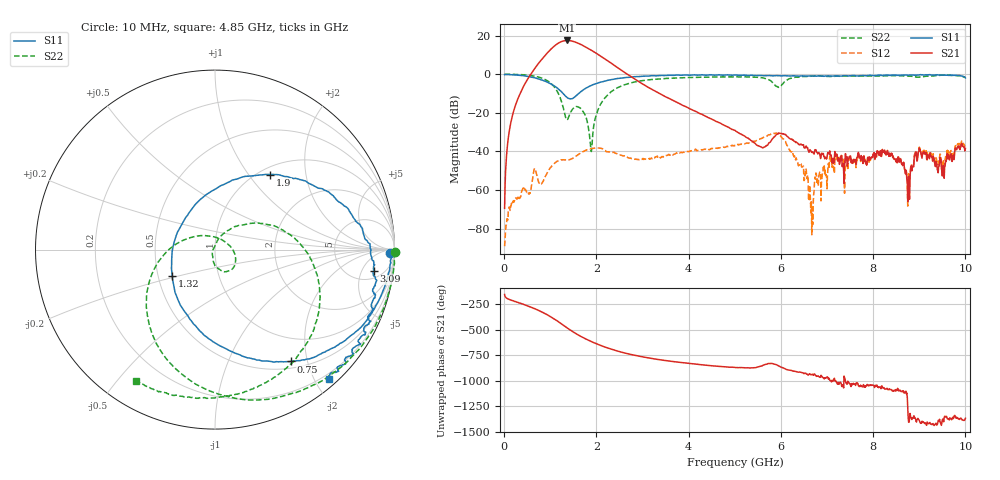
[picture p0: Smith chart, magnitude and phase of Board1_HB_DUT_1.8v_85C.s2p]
! Created Tue May 27 14:05:51 2025
# hz S ma R 50
! 2 Port Network Data from SP1.SP block
! freq  magS11  angS11  magS21  angS21  magS12  angS12  magS22  angS22
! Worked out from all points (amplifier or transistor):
!   1000 points, 10 MHz to 10 GHz, reference 50 ohm
!   highest |S21| = 17.5 dB at 1.36 GHz (marker M1)
!   |S21| within 3 dB of that: 1.083 GHz to 1.738 GHz (654.7 MHz wide, 46.4 % of centre)
!   unconditionally stable (mu >= 1): 58.74 MHz to 62.22 MHz; 90.51 MHz to 103.4 MHz; 116.1 MHz to end of sweep
!   at 1.67 GHz: K = 7.98, MAG = 16.0 dB, |S12| = -40.7 dB
!   at 5.01 GHz: K = 20.73, MAG = -12.3 dB, |S12| = -36.9 dB
!   at 10 GHz: K = 327.95, MAG = -28.9 dB, |S12| = -37.0 dB
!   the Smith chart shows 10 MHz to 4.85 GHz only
!   S11 on the Smith chart (normalised r, x): 10 MHz: 52, -44; 750 MHz: 0.60, -1.72; 1.32 GHz: 0.59, -0.19; 1.9 GHz: 1.12, +1.28; 3.09 GHz: 7, -9; 4.85 GHz: 0.12, -2.21
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1e7  0.978 -1.1  0.0003363 -153.0  3.516e-05 -168.1  1.005 -0.8
2e8  0.9631 -13.9  0.1046 145.3  0.0005206 73.5  0.9955 -18.4
7.5e8  0.7527 -55.9  1.932 50.2  0.001561 69.5  0.8425 -80.9
9.3e8  0.6291 -73.4  3.508 9.9  0.002721 115.5  0.685 -110.6
1.09e9  0.4969 -94.2  5.38 -33.2  0.004883 101.5  0.4638 -145.4
1.22e9  0.3711 -119.8  6.817 -73.2  0.005967 84.6  0.236 175.8
1.32e9  0.2793 -148.5  7.422 -105.3  0.006048 76.4  0.08705 118.4
1.36e9  0.2504 -164.8  7.493 -118.1  0.006018 75.2  0.06545 68.5
1.51e9  0.2452 128.5  7.018 -163.2  0.006941 76.3  0.1336 -31.8
1.68e9  0.3651 82.5  5.761 152.5  0.009411 67.5  0.1232 -73.0
1.9e9  0.5192 53.7  4.107 104.0  0.01188 44.8  0.01195 115.6
2.24e9  0.6914 28.9  2.239 43.9  0.009787 11.8  0.2862 31.0
2.58e9  0.8053 11.0  1.179 -2.2  0.007681 0.7  0.5186 -2.6
3.09e9  0.8927 -7.7  0.4828 -50.9  0.006394 11.3  0.7071 -38.5
3.34e9  0.9171 -15.4  0.3279 -69.3  0.0067 9.8  0.7543 -52.9
4.85e9  0.9598 -48.6  0.04273 -143.6  0.01336 -9.3  0.8534 -120.9
5.01e9  0.9597 -52.1  0.03467 -148.2  0.01423 -12.8  0.8552 -126.9
5.95e9  0.9113 -72.1  0.02999 -130.7  0.02889 -102.2  0.4559 -148.4
6.67e9  0.8992 -92.4  0.009443 142.2  6.941e-05 173.5  0.8984 -157.8
8.34e9  0.9329 -134.9  0.007466 -5.8  0.007899 -11.8  0.9142 166.9
8.75e9  0.9497 -142.1  0.0004995 174.6  0.000384 129.8  0.901 158.6
1e10  0.7998 -161.4  0.01193 74.2  0.01419 71.4  0.8321 145.3
